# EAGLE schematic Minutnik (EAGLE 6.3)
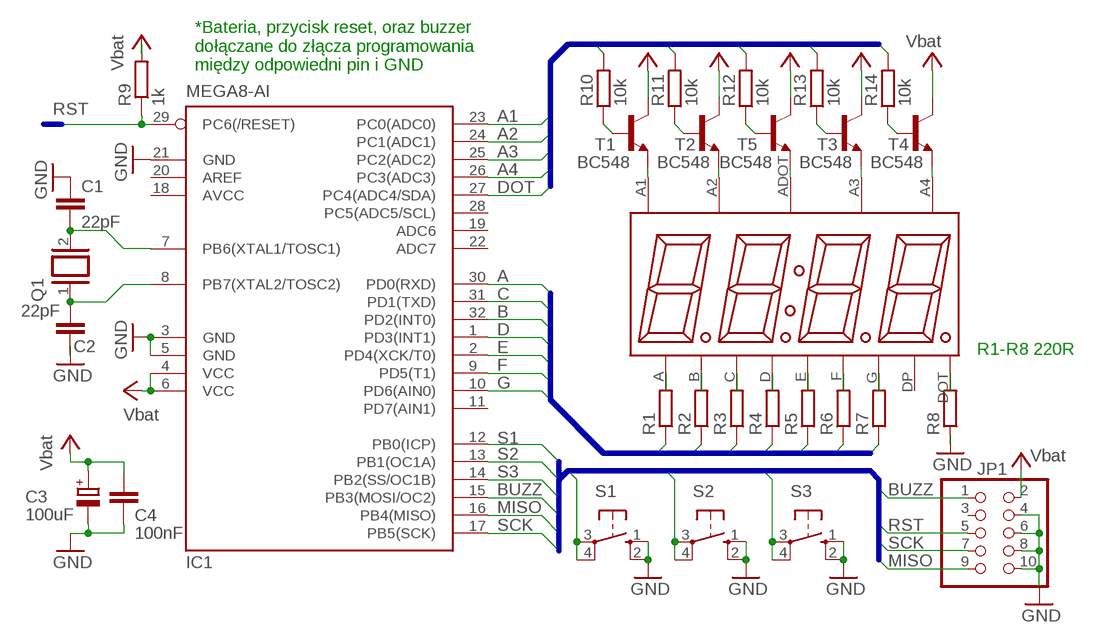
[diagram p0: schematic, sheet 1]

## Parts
C1  22pF  C-EUC0805  [C0805]
C2  22pF  C-EUC0805  [C0805]
C3  100uF  CPOL-EUE2.5-6  [E2,5-6]
C4  100nF  C-EU050-025X075  [C050-025X075]
IC1  MEGA8-AI  [TQFP32-08]
JP1  PINHD-2X5  [2X05]
Q1  XTAL/S  [QS]
R1  R-EU_0204/5  [0204/5]
R2  R-EU_0204/5  [0204/5]
R3  R-EU_0204/5  [0204/5]
R4  R-EU_0204/5  [0204/5]
R5  R-EU_0204/5  [0204/5]
R6  R-EU_0204/5  [0204/5]
R7  R-EU_0204/5  [0204/5]
R8  R-EU_0204/5  [0204/5]
R9  1k  R-EU_0204/5  [0204/5]
R10  10k  R-EU_0204/5  [0204/5]
R11  10k  R-EU_0204/5  [0204/5]
R12  10k  R-EU_0204/5  [0204/5]
R13  10k  R-EU_0204/5  [0204/5]
R14  10k  R-EU_0204/5  [0204/5]
S1  10-XX  [B3F-10XX]
S2  10-XX  [B3F-10XX]
S3  10-XX  [B3F-10XX]
T1  BC548  BC548B  [TO92-EBC]
T2  BC548  BC548B  [TO92-EBC]
T3  BC548  BC548B  [TO92-EBC]
T4  BC548  BC548B  [TO92-EBC]
T5  BC548  BC548B  [TO92-EBC]
U$1  TOF-5462DX  [TOF-5462DX]

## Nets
+5V: C3.+ C4.1 IC1.4(VCC) IC1.6(VCC) JP1.2 R9.2 T1.C T2.C T3.C T4.C T5.C ; supply symbol labelled Vbat
A: IC1.30(PD0(RXD)) R1.1
A1: IC1.23(PC0(ADC0)) R10.2
A2: IC1.24(PC1(ADC1)) R11.2
A3: IC1.25(PC2(ADC2)) R13.2
A4: IC1.26(PC3(ADC3)) R14.2
B: IC1.32(PD2(INT0)) R2.1
BUZZ: IC1.15(PB3(MOSI/OC2)) JP1.1
C: IC1.31(PD1(TXD)) R3.1
D: IC1.1(PD3(INT1)) R4.1
DOT: IC1.27(PC4(ADC4/SDA)) R12.2
E: IC1.2(PD4(XCK/T0)) R5.1
F: IC1.9(PD5(T1)) R6.1
G: IC1.10(PD6(AIN0)) R7.1
GND: C1.1 C2.1 C3.- C4.2 IC1.3(GND) IC1.5(GND) IC1.21(GND) JP1.4 JP1.6 JP1.8 JP1.10 R8.1 S1.1(S) S1.2(S1) S2.1(S) S2.2(S1) S3.1(S) S3.2(S1)
MISO: IC1.16(PB4(MISO)) JP1.9
N$1: T1.E U$1.A1
N$2: T2.E U$1.A2
N$3: T5.E U$1.ADOT
N$4: T3.E U$1.A3
N$5: T4.E U$1.A4
N$6: R1.2 U$1.A
N$7: R2.2 U$1.B
N$8: R3.2 U$1.C
N$9: R4.2 U$1.D
N$10: R5.2 U$1.E
N$11: R6.2 U$1.F
N$12: R7.2 U$1.G
N$13: R8.2 U$1.DOT
N$14: C1.2 IC1.7(PB6(XTAL1/TOSC1)) Q1.2
N$15: C2.2 IC1.8(PB7(XTAL2/TOSC2)) Q1.1
N$17: R14.1 T4.B
N$18: R13.1 T3.B
N$19: R12.1 T5.B
N$20: R11.1 T2.B
N$21: R10.1 T1.B
RST: IC1.29(PC6(/RESET)) JP1.5 R9.1
S1: IC1.12(PB0(ICP)) S1.3(P) S1.4(P1)
S2: IC1.13(PB1(OC1A)) S2.3(P) S2.4(P1)
S3: IC1.14(PB2(SS/OC1B)) S3.3(P) S3.4(P1)
SCK: IC1.17(PB5(SCK)) JP1.7
Unconnected: IC1.11(PD7(AIN1)) IC1.19(ADC6) IC1.20(AREF) IC1.22(ADC7) IC1.28(PC5(ADC5/SCL)) JP1.3 U$1.DP

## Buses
A,B,C,D,E,F,G
A1,A2,A3,A4,DOT
S1,S2,S3,BUZZ,MISO,SCK,RST

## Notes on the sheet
- *Bateria, przycisk reset, oraz buzzer
  dołączane do złącza programowania
  między odpowiedni pin i GND
- R1-R8 220R

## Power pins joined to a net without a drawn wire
AVCC: IC1.18(AVCC)

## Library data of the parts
C1 C2 C4 = rcl:C-EU: CAPACITOR, European symbol
C3 = rcl:CPOL-EU: POLARIZED CAPACITOR, European symbol
IC1 = atmel:MEGA8: MICROCONTROLLER 8 Kbytes FLASH, 1 kbytes SRAM, 512 bytes EEPROM, USART, 6-channel 10 bit ADC, 2-channel 8 bit ADC Pin compatible with Atmega48, ATMega88, ATMega168 Source: avr.lbr
JP1 = pinhead:PINHD-2X5: PIN HEADER
Q1 = special:XTAL/S: CRYSTAL
R1-R14 = rcl:R-EU_: RESISTOR, European symbol
S1-S3 = switch-omron:10-XX: OMRON SWITCH
T1-T5 = transistor-npn:BC548*: NPN Transistor
U$1 = 7seg led disp:TOF-5462DX: 7 seg multiplexed led display with common anode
